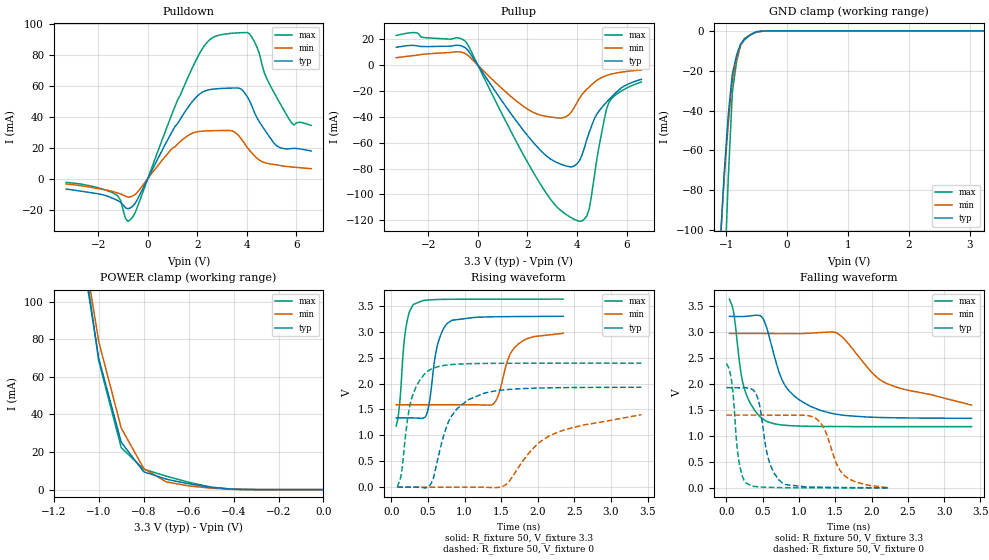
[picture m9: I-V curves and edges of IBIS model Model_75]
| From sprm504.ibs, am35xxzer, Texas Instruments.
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| Model based on original model for BC1833DV40CTPBFHP18LL_7LM_X50
|   Sub model LM_X50_PD_PU_OFF_3P3
[model]   Model_75
|[Description]  3.3V-I/O-PI-X
|[Input Load]   PI
|[Output Drive]
|Voltage   3.3V
|Mode   I/O
Model_type   I/O
Polarity   Non-Inverting
Enable   Active-Low
Vinl =  0.8V
Vinh =  2V
Cref =  15pF
Rref =  100.0000M
Vref =  0V
Vmeas =  1.65
C_comp   1.943144p   1.721292p   2.064363p
[Model Spec]
Vinl   0.8V   0.8V   0.8V
Vinh   2V   2V   2V
[Temperature Range]   25   125   -40
[Voltage Range]   3.3   2.97   3.63
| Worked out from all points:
|   slope of the pulldown table from 0 to 0.495 V, typ, clamps not added: 31.5 ohm
|   slope of the pullup table from 0 to 0.495 V, typ, clamps not added: 34.6 ohm
|   GND clamp passes 1 mA (typ) near -0.54 V on its own axis
|   POWER clamp passes 1 mA (typ) near -0.48 V on its own axis
|   rising waveform, R_fixture 50, V_fixture 3.3: 20-80 % time 137ps typ, 202ps min, 89.3ps max; typ from 1.34 V to 3.3 V
|   rising waveform, R_fixture 50, V_fixture 0: 20-80 % time 312ps typ, 707ps min, 175ps max; typ from 0 V to 1.93 V
|   falling waveform, R_fixture 50, V_fixture 3.3: 20-80 % time 379ps typ, 813ps min, 191ps max; typ from 3.3 V to 1.34 V
|   falling waveform, R_fixture 50, V_fixture 0: 20-80 % time 158ps typ, 244ps min, 92.7ps max; typ from 1.93 V to 0 V
[POWER_clamp]
-3.3V     2.432A     2.868A     2.62A
-1.067V   120.4mA    127.8mA    125.3mA
-1.033V   95.07mA    103.2mA    96.84mA
-1V       69.76mA    78.68mA    68.35mA
-900mV    25.18mA    32.74mA    22.3mA
-800mV    9.485mA    11.26mA    10.87mA
-700mV    5.568mA    4.099mA    7.163mA
-600mV    3.121mA    1.985mA    3.929mA
-500mV    1.172mA    751.7uA    1.314mA
-400mV    187uA      155.3uA    145.6uA
0V        9.358nA    43.99nA    36.65nA
[Pulldown]
-3.3V     -6.73mA    -3.436mA   -2.446mA
-1.3V     -13.54mA   -8.893mA   -10.15mA
-900mV    -18.86mA   -11.4mA    -25.9mA
-700mV    -18.91mA   -11.82mA   -26.47mA
1V        30.96mA    19.89mA    42.74mA
1.9V      51.83mA    29.94mA    75.14mA
2.9V      58.3mA     31.12mA    92.92mA
3.5V      58.67mA    30.17mA    94.2mA
4.1V      50.73mA    18.46mA    93.88mA
5.1V      22.94mA    9.149mA    55.64mA
5.8V      19.5mA     7.56mA     36.23mA
6.6V      17.91mA    6.449mA    34.47mA
[Pullup]
-3.3V     13.88mA    5.843mA    23.08mA
-2.5V     15.16mA    7.729mA    25.2mA
-500mV    13.47mA    8.991mA    18.39mA
1.4V      -39.27mA   -25.27mA   -53.66mA
2.4V      -63.29mA   -37.81mA   -88.19mA
3.5V      -77.61mA   -40.33mA   -114.8mA
4.1V      -73.95mA   -25.59mA   -120.8mA
4.5V      -51.77mA   -16.71mA   -110.8mA
4.9V      -35.15mA   -10.47mA   -62.03mA
5.2V      -28.48mA   -7.948mA   -33.38mA
5.3V      -26.46mA   -7.311mA   -28.43mA
6.6V      -10.91mA   -3.736mA   -12.96mA
[GND_clamp]
-3.3V     -2.048A    -1.805A    -3.667A
-1.1V     -108.6mA   -106.5mA   -191.4mA
-1.033V   -71.11mA   -74.03mA   -127.7mA
-966.7mV  -42.16mA   -46.82mA   -74.24mA
-900mV    -21.73mA   -24.87mA   -31.1mA
-833.3mV  -12.58mA   -14.46mA   -16.07mA
-766.7mV  -6.686mA   -7.459mA   -7.225mA
-700mV    -4.06mA    -3.869mA   -4.574mA
-566.7mV  -1.399mA   -1.472mA   -1.314mA
-500mV    -498.9uA   -685uA     -359.4uA
-300mV    -14.89uA   -26.01uA   -14.51uA
3.233V    8.831nA    14.59uA    33.57nA
[Ramp]
dV/dt_f  1.1903586/0.37664697n  0.8439098/0.80217191n  1.4763061/0.19042785n
dV/dt_r  1.1661239/0.3096566n 0.84596911/0.70409809n  1.4433969/0.17367332n
R_load = 50
[Rising Waveform]
R_fixture = 50
V_fixture = 3.3
V_fixture_min = 2.97
V_fixture_max = 3.63
67.32ps   1.337V     1.591V     1.178V
114.7ps   1.337V     1.591V     1.618V
193.9ps   1.337V     1.591V     3.024V
299.8ps   1.337V     1.591V     3.526V
487.8ps   1.429V     1.591V     3.611V
625.3ps   2.709V     1.591V     3.622V
767.9ps   3.166V     1.591V     3.626V
1.379ns   3.288V     1.592V     3.63V
1.725ns   3.294V     2.752V     3.63V
2.349ns   3.3V       2.97V      3.63V
[Rising Waveform]
R_fixture = 50
V_fixture = 0
V_fixture_min = 0
V_fixture_max = 0
81.71ps   8.754nV    123.2nV    4.04nV
137.6ps   -98.55nV   501.6nV    261.4mV
218.3ps   14.67uV    39.71nV    1.27V
277.7ps   -281.2uV   -74.17nV   1.711V
548.3ps   80.64mV    -39.9nV    2.281V
771.9ps   1.23V      50.34nV    2.359V
1.047ns   1.684V     -227.7uV   2.383V
1.553ns   1.88V      37.47mV    2.391V
2.277ns   1.92V      1.063V     2.392V
3.415ns   1.929V     1.399V     2.392V
[Falling Waveform]
R_fixture = 50
V_fixture = 3.3
V_fixture_min = 2.97
V_fixture_max = 3.63
42.74ps   3.3V       2.97V      3.63V
103.3ps   3.296V     2.97V      3.351V
235.8ps   3.295V     2.97V      1.97V
457ps     3.314V     2.97V      1.378V
548.4ps   3.112V     2.97V      1.285V
787.7ps   2.021V     2.967V     1.206V
1.15ns    1.572V     2.975V     1.184V
1.538ns   1.412V     2.964V     1.179V
2.224ns   1.35V      1.997V     1.178V
3.376ns   1.337V     1.591V     1.178V
[Falling Waveform]
R_fixture = 50
V_fixture = 0
V_fixture_min = 0
V_fixture_max = 0
0s        1.929V     1.399V     2.392V
77.49ps   1.926V     1.399V     2.003V
173.2ps   1.924V     1.399V     517.6mV
269ps     1.927V     1.399V     93.26mV
424.1ps   1.757V     1.399V     21.77mV
582.7ps   543.5mV    1.398V     10.25mV
772.2ps   93.55mV    1.398V     4.149mV
1.218ns   13.95mV    1.348V     387.7uV
1.634ns   5.857mV    230mV      46.46uV
2.248ns   8.754nV    123.2nV    4.04nV
